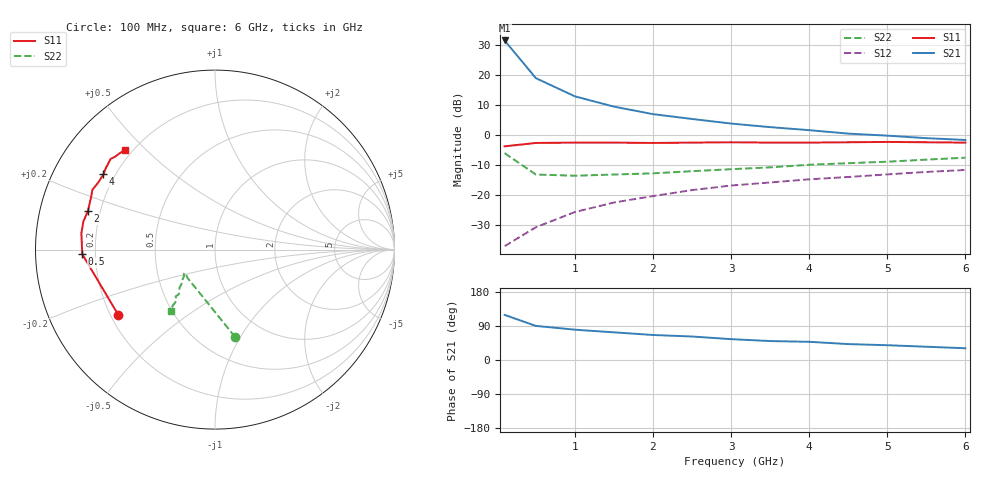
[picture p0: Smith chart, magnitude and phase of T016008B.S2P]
!AT-00600
!S-PARAMETERS at Vce=8V  Ic=60mA.  LAST UPDATED 07-21-92
# ghz s ma r 50
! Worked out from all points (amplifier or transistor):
!   13 points, 100 MHz to 6 GHz, reference 50 ohm
!   highest |S21| = 31.6 dB at 100 MHz (marker M1)
!   |S21| within 3 dB of that: start of sweep to 195.4 MHz
!   unconditionally stable (mu >= 1): 491.9 MHz to 4.845 GHz
!   at 1 GHz: K = 1.10, MAG = 17.4 dB, |S12| = -25.7 dB
!   at 3 GHz: K = 1.05, MAG = 8.9 dB, |S12| = -16.8 dB
!   at 6 GHz: K = 0.97, MSG = 5.0 dB, |S12| = -11.6 dB
!   S11 on the Smith chart (normalised r, x): 100 MHz: 0.23, -0.29; 500 MHz: 0.15, -0.02; 2 GHz: 0.15, +0.15; 4 GHz: 0.16, +0.30; 6 GHz: 0.17, +0.43
0.1  0.65 -146.0  38.06 119.0  0.014 48.0  0.5 -77.0
0.5  0.74 -178.0  8.94 90.0  0.029 65.0  0.22 -134.0
1  0.75 173.0  4.44 80.0  0.052 72.0  0.21 -142.0
1.5  0.75 168.0  2.99 73.0  0.075 76.0  0.22 -142.0
2  0.74 163.0  2.24 66.0  0.096 75.0  0.23 -139.0
2.5  0.75 157.0  1.86 62.0  0.121 76.0  0.25 -137.0
3  0.76 154.0  1.56 55.0  0.144 75.0  0.27 -134.0
3.5  0.75 150.0  1.36 50.0  0.162 75.0  0.29 -133.0
4  0.75 146.0  1.21 48.0  0.183 76.0  0.32 -129.0
4.5  0.76 143.0  1.06 42.0  0.2 74.0  0.34 -130.0
5  0.77 139.0  0.98 39.0  0.221 74.0  0.36 -127.0
5.5  0.76 137.0  0.89 35.0  0.243 73.0  0.39 -127.0
6  0.75 132.0  0.83 31.0  0.262 71.0  0.42 -126.0
